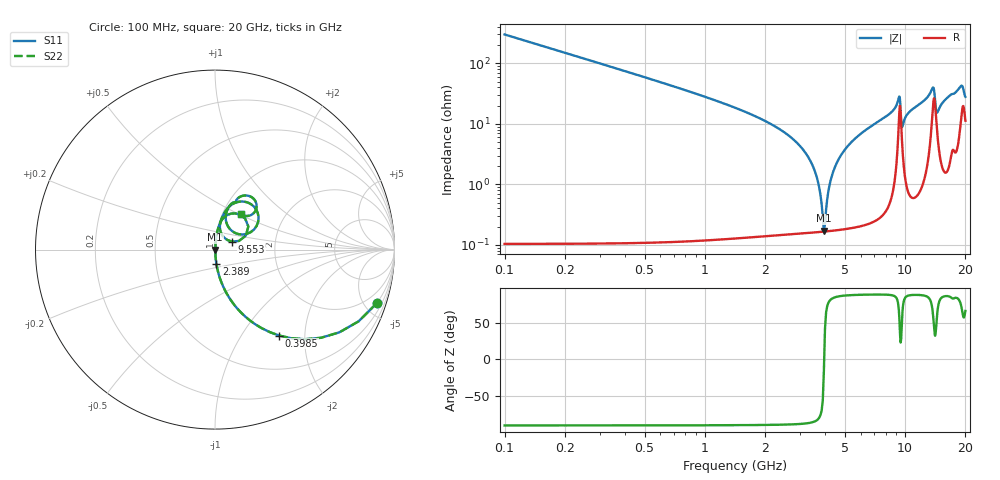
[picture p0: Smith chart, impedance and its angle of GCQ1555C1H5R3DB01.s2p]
!Murata Part Number: GCQ1555C1H5R3DB01
!These Parameters are Measured in Series Mode Connection
!Data Generated on Mar 13, 2026
!  o--ll--o
!Port1  Port2
!  o------o
!Operation Temp=25[degC], DC Bias Voltage=0[V]
!Freq. Start=100[MHz] Stop=20[GHz] 401[Steps]
# Hz S RI R 50
!Freq.(Hz) S11(Real) S11(Imag) S21(Real) S21(Imag) S12(Real) S12(Imag) S22(Real) S22(Imag)
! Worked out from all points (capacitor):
!   401 points, 100 MHz to 20 GHz, reference 50 ohm
!   read as one part in series: C = 5.3 pF near 199.5 MHz
!   lowest |Z| = 172 mohm at 3.931 GHz (marker M1)
!   series resonance near 3.942 GHz, so ESL is about 310 pH
!   S11 on the Smith chart (normalised r, x): 100 MHz: 1.00, -6.00; 398.5 MHz: 1.00, -1.49; 2.389 GHz: 1.00, -0.16; 9.553 GHz: 1.21, +0.11; 20 GHz: 1.23, +0.51
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1e8  0.9 -0.2999  0.1 0.2999  0.1 0.2999  0.9 -0.2999
3.985e8  0.3576 -0.4786  0.6424 0.4786  0.6424 0.4786  0.3576 -0.4786
9.4575e8  0.0831 -0.2741  0.9169 0.2741  0.9169 0.2741  0.0831 -0.2741
2.3885e9  0.00775 -0.0791  0.9922 0.0791  0.9922 0.0791  0.00775 -0.0791
3.43325e9  0.00204 -0.0212  0.998 0.0212  0.998 0.0212  0.00204 -0.0212
3.682e9  0.00174 -0.0105  0.9983 0.0105  0.9983 0.0105  0.00174 -0.0105
3.93075e9  0.00166 -0.000432  0.9983 0.000432  0.9983 0.000432  0.00166 -0.000432
4.03025e9  0.00168 0.00341  0.9983 -0.00341  0.9983 -0.00341  0.00168 0.00341
4.279e9  0.00187 0.0127  0.9981 -0.0127  0.9981 -0.0127  0.00187 0.0127
4.72675e9  0.00257 0.0282  0.9974 -0.0282  0.9974 -0.0282  0.00257 0.0282
5.52275e9  0.0048 0.0536  0.9952 -0.0536  0.9952 -0.0536  0.0048 0.0536
6.7665e9  0.0105 0.0903  0.9895 -0.0903  0.9895 -0.0903  0.0105 0.0903
9.30375e9  0.1383 0.1954  0.8617 -0.1954  0.8617 -0.1954  0.1383 0.1954
9.5525e9  0.096 0.0445  0.904 -0.0445  0.904 -0.0445  0.096 0.0445
9.70175e9  0.0428 0.0765  0.9572 -0.0765  0.9572 -0.0765  0.0428 0.0765
1.005e10  0.0272 0.1242  0.9728 -0.1242  0.9728 -0.1242  0.0272 0.1242
1.338325e10  0.1346 0.2668  0.8654 -0.2668  0.8654 -0.2668  0.1346 0.2668
1.3831e10  0.2379 0.2054  0.7621 -0.2054  0.7621 -0.2054  0.2379 0.2054
1.4428e10  0.0866 0.1111  0.9134 -0.1111  0.9134 -0.1111  0.0866 0.1111
1.67165e10  0.0963 0.2594  0.9037 -0.2594  0.9037 -0.2594  0.0963 0.2594
1.905475e10  0.2132 0.2851  0.7868 -0.2851  0.7868 -0.2851  0.2132 0.2851
2e10  0.1465 0.1966  0.8535 -0.1966  0.8535 -0.1966  0.1465 0.1966
